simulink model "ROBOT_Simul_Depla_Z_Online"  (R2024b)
settings: Solver=ode15s  StartTime=0.0  StopTime=0.2  RelTol=1e-3  EnableMultiTasking=on
undefined symbols (not defined in the file): BATI1_Défaut_sldprt, BATI2_Défaut_sldprt, BATI3_Défaut_sldprt, BIELLE_Défaut_sldprt, BRAS_Défaut_sldprt, deg, Drive, EFFECTEUR_Défaut_sldprt, Fichiers, Fichiers_Matlab_sujetB, JOINT_Défaut_sldprt, kg, m, MANETTE_Défaut_sldprt, MATLAB, Matlab, mm, N, PIED_Défaut_sldprt, rad, s, STL, X, Y, Z
libraries: sm_lib x139, fl_lib x42, nesl_utility x19, slpidlib x3
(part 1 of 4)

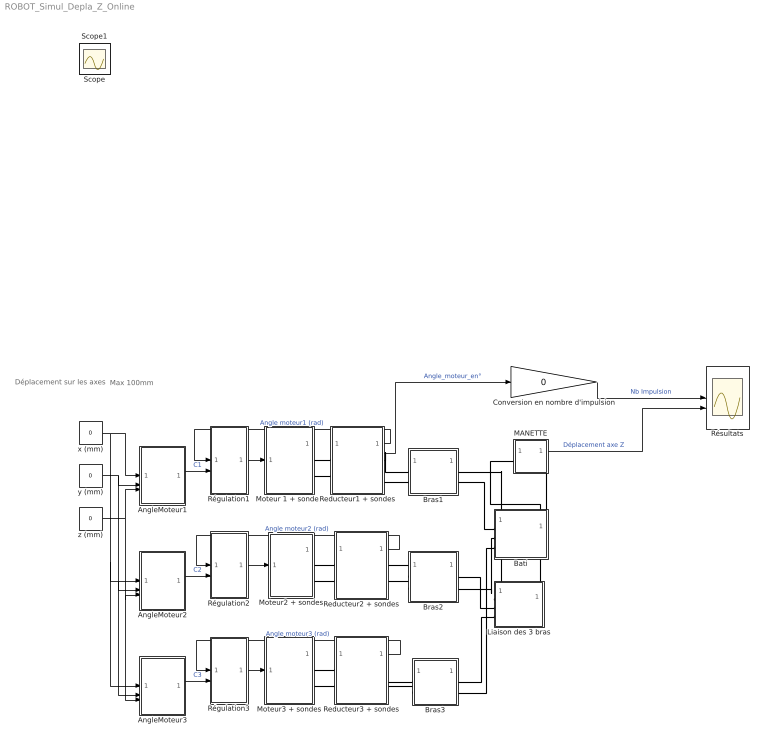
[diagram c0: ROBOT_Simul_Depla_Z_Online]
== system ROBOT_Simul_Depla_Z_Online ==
  note: Déplacement sur les axes
  note: Max 100mm
  AngleMoteur1 : MATLAB Function  TreatAsAtomicUnit=on
  AngleMoteur2 : MATLAB Function  TreatAsAtomicUnit=on
  AngleMoteur3 : MATLAB Function  TreatAsAtomicUnit=on
  Bati : Subsystem
  Bras1 : Subsystem
  Bras2 : Subsystem
  Bras3 : Subsystem
  Conversion en nombre d'impulsion : Gain  Gain=0
  Liaison des 3 bras : Subsystem
  MANETTE : Subsystem
  Moteur 1 + sondes : Subsystem
  Moteur2 + sondes : Subsystem
  Moteur3 + sondes : Subsystem
  Reducteur1 + sondes : Subsystem
  Reducteur2 + sondes : Subsystem
  Reducteur3 + sondes : Subsystem
  Régulation1 : Subsystem
  Régulation2 : Subsystem
  Régulation3 : Subsystem
  Résultats : Scope  NumInputPorts=2
  x (mm) : Constant  Value=0
  y (mm) : Constant  Value=0
  z (mm) : Constant  Value=0
  Scope : Scope
  Scope1 : Scope
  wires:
  Régulation3/1(Out1) -> Moteur3 + sondes/1(In1)
  Reducteur3 + sondes/1(Angle_mot3) -> Régulation3/1(In1)  "Angle moteur3 (rad)"
  Régulation1/1(Out1) -> Moteur 1 + sondes/1(In1)
  Reducteur1 + sondes/1(Angle_mot1) -> Régulation1/1(In1)  "Angle moteur1 (rad)"
  Régulation2/1(Out1) -> Moteur2 + sondes/1(In1)
  Reducteur2 + sondes/1(Angle_mot2) -> Régulation2/1(In1)  "Angle moteur2 (rad)"
  AngleMoteur3/1(anglmot3) -> Régulation3/2(In2)  "C3"
  x (mm)/1 -> AngleMoteur1/1(x), AngleMoteur2/1(x), AngleMoteur3/1(x)
  AngleMoteur1/1(anglmot1) -> Régulation1/2(In2)  "C1"
  AngleMoteur2/1(anglmot2) -> Régulation2/2(In2)  "C2"
  y (mm)/1 -> AngleMoteur1/2(y), AngleMoteur2/2(y), AngleMoteur3/2(y)
  z (mm)/1 -> AngleMoteur1/3(z), AngleMoteur2/3(z), AngleMoteur3/3(z)
  Reducteur1 + sondes/2(Angle_mot_°) -> Conversion en nombre d'impulsion/1  "Angle_moteur_en°"
  Conversion en nombre d'impulsion/1 -> Résultats/1  "Nb Impulsion"
  MANETTE/1(Out1) -> Résultats/2  "Déplacement axe Z"
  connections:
  Liaison des 3 bras/RConn1 -- MANETTE/LConn1
  Moteur3 + sondes/RConn1 -- Reducteur3 + sondes/LConn1
  Moteur 1 + sondes/RConn1 -- Reducteur1 + sondes/LConn1
  Moteur3 + sondes/RConn2 -- Reducteur3 + sondes/LConn2
  Reducteur1 + sondes/LConn2 -- Moteur 1 + sondes/RConn2
  Moteur2 + sondes/RConn2 -- Reducteur2 + sondes/LConn2
  Moteur2 + sondes/RConn1 -- Reducteur2 + sondes/LConn1
  Reducteur1 + sondes/RConn1 -- Bras1/LConn1
  Reducteur1 + sondes/RConn2 -- Bras1/LConn2
  Liaison des 3 bras/LConn1 -- Bras1/RConn1
  Liaison des 3 bras/LConn2 -- Bras2/RConn1
  Bras2/LConn1 -- Reducteur2 + sondes/RConn1
  Bras2/LConn2 -- Reducteur2 + sondes/RConn2
  Liaison des 3 bras/LConn3 -- Bras3/RConn1
  Reducteur3 + sondes/RConn1 -- Bras3/LConn1
  Bras3/LConn2 -- Reducteur3 + sondes/RConn2
  Bati/LConn1 -- Bras1/RConn2
  Bati/LConn2 -- Bras2/RConn2
  Bati/LConn3 -- Bras3/RConn2
  MANETTE/RConn1 -- Bati/RConn1

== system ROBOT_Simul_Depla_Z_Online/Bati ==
  BATI_1_RIGID : Subsystem
  MechanismConfiguration : sm_lib/Utilities/Mechanism Configuration  UniformGravity=Constant  GravityVector=[0 -9.81 0]  GravityVectorUnits=m/s^2  LinearizationDelta=0.001  JointModeTransitionNonlinearIterations=2
  Solver Configuration : nesl_utility/Solver Configuration  PhysicalDomain=network_engine_domain  SubClassName=solver  LeftPortType=input  RightPortType=generic  Tones=[]  Harmonics=[]  SimulateNoise=off  Profile=off  UseLocalSampling=off  EnableSwitchedLinearOptims=on  FrequencyDomain=off  UseCCode=off  RelTol=0.001  AbsTol=1e-06  MinStep=1e-09  ToWorkspace=off  RevertToSquareIcSolve=off  NumHomotopyIterations=100  PhasorMode=off  PhasorModeNumHarmonics=1  ConsistencySolver=NEWTON_FTOL  IndexReductionMethod=DerivativeReplacement  DoDC=off  ResidualTolerance=1e-09  ConsistencyTolSource=GLOBAL  ConsistencyAbsTol=0.001  ConsistencyRelTol=0.001  ConsistencyTolFactor=0.001  UseLocalSolver=off  LocalSolverChoice=NE_BACKWARD_EULER_ADVANCER  ResolveIndetEquations=on  FunctionEvalNumThread=1  LocalSolverSampleTime=0.001  DoFixedCost=off  MaxNonlinIter=3  MaxModeIter=2  ComputeImpulses=off  ImpulseIterations=2  LinearAlgebra=Sparse  LinearAlgebraNumThread=0  EquationFormulation=NE_TIME_EF  DelaysMemoryBudget=1024  AutomaticFiltering=on  FilteringTimeConstant=0.001  PartitionStorageMethod=AS_NEEDED  PartitionMemoryBudget=1024  PartitionMethod=FAST  MultibodyUseLocalSolver=off  MultibodyLocalSolverChoice=ODE1  MultibodyLocalSolverSampleTime=0.001
  Transform : sm_lib/Frames and Transforms/Rigid Transform  RotationMethod=ArbitraryAxis  FollAlignAxisA=+X  BaseAlignAxisA=+Y  FollAlignAxisB=+Y  BaseAlignAxisB=+Z  RotationStandardAxis=+Z  RotationAngle=1.8228218707828856  RotationAngleUnits=rad  RotationArbitraryAxis=[4.4011854841110467e-16 1.1162668393823967e-16 -1]  RotationSequenceAxes=FollowerAxes  RotationSequence=XYX  RotationSequenceAngles=[0 0 0]  RotationSequenceAnglesUnits=deg  RotationMatrix=[1 0 0; 0 1 0; 0 0 1]  Quaternion=[1 0 0 0]  TranslationMethod=Cartesian  TranslationCartesianOffset=[14.920329062241711 -30.551170260312524 -19.999999999988649]  TranslationCartesianOffsetUnits=mm  TranslationStandardAxis=+Z  TranslationStandardOffset=0  TranslationStandardOffsetUnits=mm  TranslationROffset=0  TranslationROffsetUnits=m  TranslationThetaOffset=0  TranslationThetaOffsetUnits=deg  TranslationZOffset=0  TranslationZOffsetUnits=m
  World : sm_lib/Frames and Transforms/World Frame
  E1 : PMIOPort  Side=Left
  E2 : PMIOPort  Port=2  Side=Left
  E3 : PMIOPort  Port=3  Side=Left
  Wrld : PMIOPort  Port=4  Side=Right
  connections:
  Transform/LConn1 -- MechanismConfiguration/RConn1 -- Wrld/RConn1 -- World/RConn1 -- Solver Configuration/RConn1
  BATI_1_RIGID/LConn1 -- Transform/RConn1
  BATI_1_RIGID/RConn3 -- E1/RConn1
  BATI_1_RIGID/RConn1 -- E3/RConn1
  BATI_1_RIGID/RConn2 -- E2/RConn1

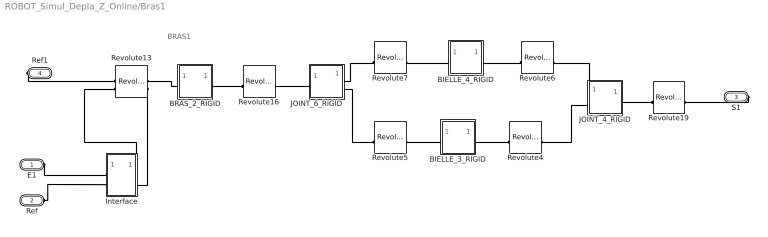
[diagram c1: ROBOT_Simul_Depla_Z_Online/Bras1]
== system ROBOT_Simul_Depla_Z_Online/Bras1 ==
  note: BRAS1
  BIELLE_3_RIGID : Subsystem
  BIELLE_4_RIGID : Subsystem
  BRAS_2_RIGID : Subsystem
  Interface : Subsystem
  JOINT_4_RIGID : Subsystem
  JOINT_6_RIGID : Subsystem
  Revolute13 : sm_lib/Joints/Revolute Joint  JointMode=Normal  CompositeWrenchDir=FollowerOnBase  CompositeWrenchFrame=BaseFrame  SenseConstraintForce=off  SenseConstraintTorque=off  SenseTotalForce=off  SenseTotalTorque=off  PositionTargetSpecify=on  PositionTargetPriority=Low  PositionTargetValue=11.887378711744704  PositionTargetValueUnits=deg  VelocityTargetSpecify=off  VelocityTargetPriority=High  VelocityTargetValue=0  VelocityTargetValueUnits=deg/s  EquilibriumPosition=0  EquilibriumPositionUnits=rad  SpringStiffness=0  SpringStiffnessUnits=m*N/rad  DampingCoefficient=0  DampingCoefficientUnits=m*s*N/rad  LowerLimitSpecify=off  LowerLimitBound=-90  LowerLimitBoundUnits=deg  LowerLimitStiffness=1e4  LowerLimitStiffnessUnits=N*m/deg  LowerLimitDamping=10  LowerLimitDampingUnits=N*m/(deg/s)  LowerLimitTransitionRegionWidth=0.1  LowerLimitTransitionRegionWidthUnits=deg  UpperLimitSpecify=off  UpperLimitBound=90  UpperLimitBoundUnits=deg  UpperLimitStiffness=1e4  UpperLimitStiffnessUnits=N*m/deg  UpperLimitDamping=10  UpperLimitDampingUnits=N*m/(deg/s)  UpperLimitTransitionRegionWidth=0.1  UpperLimitTransitionRegionWidthUnits=deg  TorqueActuationMode=InputTorque  MotionActuationMode=ComputedMotion  SensePosition=off  SenseVelocity=on  SenseAcceleration=off  SenseTorqueForce=off  SenseLowerLimitTorqueForce=off  SenseUpperLimitTorqueForce=off
  Revolute16 : sm_lib/Joints/Revolute Joint  JointMode=Normal  CompositeWrenchDir=FollowerOnBase  CompositeWrenchFrame=BaseFrame  SenseConstraintForce=off  SenseConstraintTorque=off  SenseTotalForce=off  SenseTotalTorque=off  PositionTargetSpecify=on  PositionTargetPriority=Low  PositionTargetValue=-127.14100786995047  PositionTargetValueUnits=deg  VelocityTargetSpecify=off  VelocityTargetPriority=High  VelocityTargetValue=0  VelocityTargetValueUnits=deg/s  EquilibriumPosition=0  EquilibriumPositionUnits=rad  SpringStiffness=0  SpringStiffnessUnits=m*N/rad  DampingCoefficient=0  DampingCoefficientUnits=m*s*N/rad  LowerLimitSpecify=off  LowerLimitBound=-90  LowerLimitBoundUnits=deg  LowerLimitStiffness=1e4  LowerLimitStiffnessUnits=N*m/deg  LowerLimitDamping=10  LowerLimitDampingUnits=N*m/(deg/s)  LowerLimitTransitionRegionWidth=0.1  LowerLimitTransitionRegionWidthUnits=deg  UpperLimitSpecify=off  UpperLimitBound=90  UpperLimitBoundUnits=deg  UpperLimitStiffness=1e4  UpperLimitStiffnessUnits=N*m/deg  UpperLimitDamping=10  UpperLimitDampingUnits=N*m/(deg/s)  UpperLimitTransitionRegionWidth=0.1  UpperLimitTransitionRegionWidthUnits=deg  TorqueActuationMode=NoTorque  MotionActuationMode=ComputedMotion  SensePosition=off  SenseVelocity=off  SenseAcceleration=off  SenseTorqueForce=off  SenseLowerLimitTorqueForce=off  SenseUpperLimitTorqueForce=off
  Revolute19 : sm_lib/Joints/Revolute Joint  JointMode=Normal  CompositeWrenchDir=FollowerOnBase  CompositeWrenchFrame=BaseFrame  SenseConstraintForce=off  SenseConstraintTorque=off  SenseTotalForce=off  SenseTotalTorque=off  PositionTargetSpecify=off  PositionTargetPriority=High  PositionTargetValue=0  PositionTargetValueUnits=deg  VelocityTargetSpecify=off  VelocityTargetPriority=High  VelocityTargetValue=0  VelocityTargetValueUnits=deg/s  EquilibriumPosition=0  EquilibriumPositionUnits=rad  SpringStiffness=0  SpringStiffnessUnits=m*N/rad  DampingCoefficient=0  DampingCoefficientUnits=m*s*N/rad  LowerLimitSpecify=off  LowerLimitBound=-90  LowerLimitBoundUnits=deg  LowerLimitStiffness=1e4  LowerLimitStiffnessUnits=N*m/deg  LowerLimitDamping=10  LowerLimitDampingUnits=N*m/(deg/s)  LowerLimitTransitionRegionWidth=0.1  LowerLimitTransitionRegionWidthUnits=deg  UpperLimitSpecify=off  UpperLimitBound=90  UpperLimitBoundUnits=deg  UpperLimitStiffness=1e4  UpperLimitStiffnessUnits=N*m/deg  UpperLimitDamping=10  UpperLimitDampingUnits=N*m/(deg/s)  UpperLimitTransitionRegionWidth=0.1  UpperLimitTransitionRegionWidthUnits=deg  TorqueActuationMode=NoTorque  MotionActuationMode=ComputedMotion  SensePosition=off  SenseVelocity=off  SenseAcceleration=off  SenseTorqueForce=off  SenseLowerLimitTorqueForce=off  SenseUpperLimitTorqueForce=off
  Revolute4 : sm_lib/Joints/Revolute Joint  JointMode=Normal  CompositeWrenchDir=FollowerOnBase  CompositeWrenchFrame=BaseFrame  SenseConstraintForce=off  SenseConstraintTorque=off  SenseTotalForce=off  SenseTotalTorque=off  PositionTargetSpecify=on  PositionTargetPriority=Low  PositionTargetValue=-91.30254308411611  PositionTargetValueUnits=deg  VelocityTargetSpecify=off  VelocityTargetPriority=High  VelocityTargetValue=0  VelocityTargetValueUnits=deg/s  EquilibriumPosition=0  EquilibriumPositionUnits=rad  SpringStiffness=0  SpringStiffnessUnits=m*N/rad  DampingCoefficient=0  DampingCoefficientUnits=m*s*N/rad  LowerLimitSpecify=off  LowerLimitBound=-90  LowerLimitBoundUnits=deg  LowerLimitStiffness=1e4  LowerLimitStiffnessUnits=N*m/deg  LowerLimitDamping=10  LowerLimitDampingUnits=N*m/(deg/s)  LowerLimitTransitionRegionWidth=0.1  LowerLimitTransitionRegionWidthUnits=deg  UpperLimitSpecify=off  UpperLimitBound=90  UpperLimitBoundUnits=deg  UpperLimitStiffness=1e4  UpperLimitStiffnessUnits=N*m/deg  UpperLimitDamping=10  UpperLimitDampingUnits=N*m/(deg/s)  UpperLimitTransitionRegionWidth=0.1  UpperLimitTransitionRegionWidthUnits=deg  TorqueActuationMode=NoTorque  MotionActuationMode=ComputedMotion  SensePosition=off  SenseVelocity=off  SenseAcceleration=off  SenseTorqueForce=off  SenseLowerLimitTorqueForce=off  SenseUpperLimitTorqueForce=off
  Revolute5 : sm_lib/Joints/Revolute Joint  JointMode=Normal  CompositeWrenchDir=FollowerOnBase  CompositeWrenchFrame=BaseFrame  SenseConstraintForce=off  SenseConstraintTorque=off  SenseTotalForce=off  SenseTotalTorque=off  PositionTargetSpecify=on  PositionTargetPriority=Low  PositionTargetValue=-91.302543084116394  PositionTargetValueUnits=deg  VelocityTargetSpecify=off  VelocityTargetPriority=High  VelocityTargetValue=0  VelocityTargetValueUnits=deg/s  EquilibriumPosition=0  EquilibriumPositionUnits=rad  SpringStiffness=0  SpringStiffnessUnits=m*N/rad  DampingCoefficient=0  DampingCoefficientUnits=m*s*N/rad  LowerLimitSpecify=off  LowerLimitBound=-90  LowerLimitBoundUnits=deg  LowerLimitStiffness=1e4  LowerLimitStiffnessUnits=N*m/deg  LowerLimitDamping=10  LowerLimitDampingUnits=N*m/(deg/s)  LowerLimitTransitionRegionWidth=0.1  LowerLimitTransitionRegionWidthUnits=deg  UpperLimitSpecify=off  UpperLimitBound=90  UpperLimitBoundUnits=deg  UpperLimitStiffness=1e4  UpperLimitStiffnessUnits=N*m/deg  UpperLimitDamping=10  UpperLimitDampingUnits=N*m/(deg/s)  UpperLimitTransitionRegionWidth=0.1  UpperLimitTransitionRegionWidthUnits=deg  TorqueActuationMode=NoTorque  MotionActuationMode=ComputedMotion  SensePosition=off  SenseVelocity=off  SenseAcceleration=off  SenseTorqueForce=off  SenseLowerLimitTorqueForce=off  SenseUpperLimitTorqueForce=off
  Revolute6 : sm_lib/Joints/Revolute Joint  JointMode=Normal  CompositeWrenchDir=FollowerOnBase  CompositeWrenchFrame=BaseFrame  SenseConstraintForce=off  SenseConstraintTorque=off  SenseTotalForce=off  SenseTotalTorque=off  PositionTargetSpecify=off  PositionTargetPriority=High  PositionTargetValue=0  PositionTargetValueUnits=deg  VelocityTargetSpecify=off  VelocityTargetPriority=High  VelocityTargetValue=0  VelocityTargetValueUnits=deg/s  EquilibriumPosition=0  EquilibriumPositionUnits=rad  SpringStiffness=0  SpringStiffnessUnits=m*N/rad  DampingCoefficient=0  DampingCoefficientUnits=m*s*N/rad  LowerLimitSpecify=off  LowerLimitBound=-90  LowerLimitBoundUnits=deg  LowerLimitStiffness=1e4  LowerLimitStiffnessUnits=N*m/deg  LowerLimitDamping=10  LowerLimitDampingUnits=N*m/(deg/s)  LowerLimitTransitionRegionWidth=0.1  LowerLimitTransitionRegionWidthUnits=deg  UpperLimitSpecify=off  UpperLimitBound=90  UpperLimitBoundUnits=deg  UpperLimitStiffness=1e4  UpperLimitStiffnessUnits=N*m/deg  UpperLimitDamping=10  UpperLimitDampingUnits=N*m/(deg/s)  UpperLimitTransitionRegionWidth=0.1  UpperLimitTransitionRegionWidthUnits=deg  TorqueActuationMode=NoTorque  MotionActuationMode=ComputedMotion  SensePosition=off  SenseVelocity=off  SenseAcceleration=off  SenseTorqueForce=off  SenseLowerLimitTorqueForce=off  SenseUpperLimitTorqueForce=off
  Revolute7 : sm_lib/Joints/Revolute Joint  JointMode=Normal  CompositeWrenchDir=FollowerOnBase  CompositeWrenchFrame=BaseFrame  SenseConstraintForce=off  SenseConstraintTorque=off  SenseTotalForce=off  SenseTotalTorque=off  PositionTargetSpecify=on  PositionTargetPriority=Low  PositionTargetValue=91.302543084116408  PositionTargetValueUnits=deg  VelocityTargetSpecify=off  VelocityTargetPriority=High  VelocityTargetValue=0  VelocityTargetValueUnits=deg/s  EquilibriumPosition=0  EquilibriumPositionUnits=rad  SpringStiffness=0  SpringStiffnessUnits=m*N/rad  DampingCoefficient=0  DampingCoefficientUnits=m*s*N/rad  LowerLimitSpecify=off  LowerLimitBound=-90  LowerLimitBoundUnits=deg  LowerLimitStiffness=1e4  LowerLimitStiffnessUnits=N*m/deg  LowerLimitDamping=10  LowerLimitDampingUnits=N*m/(deg/s)  LowerLimitTransitionRegionWidth=0.1  LowerLimitTransitionRegionWidthUnits=deg  UpperLimitSpecify=off  UpperLimitBound=90  UpperLimitBoundUnits=deg  UpperLimitStiffness=1e4  UpperLimitStiffnessUnits=N*m/deg  UpperLimitDamping=10  UpperLimitDampingUnits=N*m/(deg/s)  UpperLimitTransitionRegionWidth=0.1  UpperLimitTransitionRegionWidthUnits=deg  TorqueActuationMode=NoTorque  MotionActuationMode=ComputedMotion  SensePosition=off  SenseVelocity=off  SenseAcceleration=off  SenseTorqueForce=off  SenseLowerLimitTorqueForce=off  SenseUpperLimitTorqueForce=off
  E1 : PMIOPort  Side=Left
  Ref : PMIOPort  Port=2  Side=Left
  S1 : PMIOPort  Port=3  Side=Right
  Ref1 : PMIOPort  Port=4  Side=Right
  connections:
  JOINT_4_RIGID/LConn2 -- Revolute4/RConn1
  BIELLE_4_RIGID/LConn1 -- Revolute7/LConn1
  BIELLE_3_RIGID/LConn1 -- Revolute5/LConn1
  JOINT_6_RIGID/RConn2 -- Revolute5/RConn1
  BIELLE_4_RIGID/RConn1 -- Revolute6/LConn1
  JOINT_4_RIGID/LConn1 -- Revolute6/RConn1
  BRAS_2_RIGID/RConn1 -- Revolute16/LConn1
  S1/RConn1 -- Revolute19/LConn1
  BRAS_2_RIGID/LConn1 -- Revolute13/RConn1
  JOINT_4_RIGID/RConn1 -- Revolute19/RConn1
  JOINT_6_RIGID/LConn1 -- Revolute16/RConn1
  Ref1/RConn1 -- Revolute13/LConn1
  JOINT_6_RIGID/RConn1 -- Revolute7/RConn1
  BIELLE_3_RIGID/RConn1 -- Revolute4/LConn1
  Interface/RConn1 -- Revolute13/LConn2
  Interface/RConn2 -- Revolute13/RConn2
  E1/RConn1 -- Interface/LConn1
  Ref/RConn1 -- Interface/LConn2

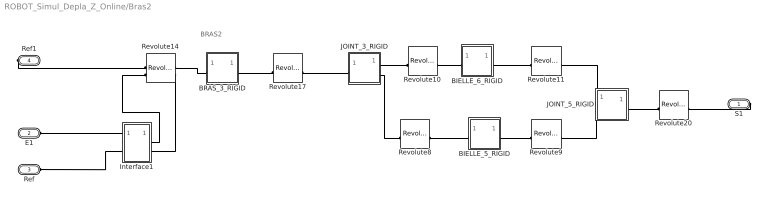
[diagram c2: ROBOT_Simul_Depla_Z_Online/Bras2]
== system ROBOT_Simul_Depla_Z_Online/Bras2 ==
  note: BRAS2
  BIELLE_5_RIGID : Subsystem
  BIELLE_6_RIGID : Subsystem
  BRAS_3_RIGID : Subsystem
  Interface1 : Subsystem
  JOINT_3_RIGID : Subsystem
  JOINT_5_RIGID : Subsystem
  Revolute10 : sm_lib/Joints/Revolute Joint  JointMode=Normal  CompositeWrenchDir=FollowerOnBase  CompositeWrenchFrame=BaseFrame  SenseConstraintForce=off  SenseConstraintTorque=off  SenseTotalForce=off  SenseTotalTorque=off  PositionTargetSpecify=on  PositionTargetPriority=Low  PositionTargetValue=-88.697456915883507  PositionTargetValueUnits=deg  VelocityTargetSpecify=off  VelocityTargetPriority=High  VelocityTargetValue=0  VelocityTargetValueUnits=deg/s  EquilibriumPosition=0  EquilibriumPositionUnits=rad  SpringStiffness=0  SpringStiffnessUnits=m*N/rad  DampingCoefficient=0  DampingCoefficientUnits=m*s*N/rad  LowerLimitSpecify=off  LowerLimitBound=-90  LowerLimitBoundUnits=deg  LowerLimitStiffness=1e4  LowerLimitStiffnessUnits=N*m/deg  LowerLimitDamping=10  LowerLimitDampingUnits=N*m/(deg/s)  LowerLimitTransitionRegionWidth=0.1  LowerLimitTransitionRegionWidthUnits=deg  UpperLimitSpecify=off  UpperLimitBound=90  UpperLimitBoundUnits=deg  UpperLimitStiffness=1e4  UpperLimitStiffnessUnits=N*m/deg  UpperLimitDamping=10  UpperLimitDampingUnits=N*m/(deg/s)  UpperLimitTransitionRegionWidth=0.1  UpperLimitTransitionRegionWidthUnits=deg  TorqueActuationMode=NoTorque  MotionActuationMode=ComputedMotion  SensePosition=off  SenseVelocity=off  SenseAcceleration=off  SenseTorqueForce=off  SenseLowerLimitTorqueForce=off  SenseUpperLimitTorqueForce=off
  Revolute11 : sm_lib/Joints/Revolute Joint  JointMode=Normal  CompositeWrenchDir=FollowerOnBase  CompositeWrenchFrame=BaseFrame  SenseConstraintForce=off  SenseConstraintTorque=off  SenseTotalForce=off  SenseTotalTorque=off  PositionTargetSpecify=off  PositionTargetPriority=High  PositionTargetValue=0  PositionTargetValueUnits=deg  VelocityTargetSpecify=off  VelocityTargetPriority=High  VelocityTargetValue=0  VelocityTargetValueUnits=deg/s  EquilibriumPosition=0  EquilibriumPositionUnits=rad  SpringStiffness=0  SpringStiffnessUnits=m*N/rad  DampingCoefficient=0  DampingCoefficientUnits=m*s*N/rad  LowerLimitSpecify=off  LowerLimitBound=-90  LowerLimitBoundUnits=deg  LowerLimitStiffness=1e4  LowerLimitStiffnessUnits=N*m/deg  LowerLimitDamping=10  LowerLimitDampingUnits=N*m/(deg/s)  LowerLimitTransitionRegionWidth=0.1  LowerLimitTransitionRegionWidthUnits=deg  UpperLimitSpecify=off  UpperLimitBound=90  UpperLimitBoundUnits=deg  UpperLimitStiffness=1e4  UpperLimitStiffnessUnits=N*m/deg  UpperLimitDamping=10  UpperLimitDampingUnits=N*m/(deg/s)  UpperLimitTransitionRegionWidth=0.1  UpperLimitTransitionRegionWidthUnits=deg  TorqueActuationMode=NoTorque  MotionActuationMode=ComputedMotion  SensePosition=off  SenseVelocity=off  SenseAcceleration=off  SenseTorqueForce=off  SenseLowerLimitTorqueForce=off  SenseUpperLimitTorqueForce=off
  Revolute14 : sm_lib/Joints/Revolute Joint  JointMode=Normal  CompositeWrenchDir=FollowerOnBase  CompositeWrenchFrame=BaseFrame  SenseConstraintForce=off  SenseConstraintTorque=off  SenseTotalForce=off  SenseTotalTorque=off  PositionTargetSpecify=on  PositionTargetPriority=Low  PositionTargetValue=-168.11262128825132  PositionTargetValueUnits=deg  VelocityTargetSpecify=off  VelocityTargetPriority=High  VelocityTargetValue=0  VelocityTargetValueUnits=deg/s  EquilibriumPosition=0  EquilibriumPositionUnits=rad  SpringStiffness=0  SpringStiffnessUnits=m*N/rad  DampingCoefficient=0  DampingCoefficientUnits=m*s*N/rad  LowerLimitSpecify=off  LowerLimitBound=-90  LowerLimitBoundUnits=deg  LowerLimitStiffness=1e4  LowerLimitStiffnessUnits=N*m/deg  LowerLimitDamping=10  LowerLimitDampingUnits=N*m/(deg/s)  LowerLimitTransitionRegionWidth=0.1  LowerLimitTransitionRegionWidthUnits=deg  UpperLimitSpecify=off  UpperLimitBound=90  UpperLimitBoundUnits=deg  UpperLimitStiffness=1e4  UpperLimitStiffnessUnits=N*m/deg  UpperLimitDamping=10  UpperLimitDampingUnits=N*m/(deg/s)  UpperLimitTransitionRegionWidth=0.1  UpperLimitTransitionRegionWidthUnits=deg  TorqueActuationMode=InputTorque  MotionActuationMode=ComputedMotion  SensePosition=off  SenseVelocity=on  SenseAcceleration=off  SenseTorqueForce=off  SenseLowerLimitTorqueForce=off  SenseUpperLimitTorqueForce=off
  Revolute17 : sm_lib/Joints/Revolute Joint  JointMode=Normal  CompositeWrenchDir=FollowerOnBase  CompositeWrenchFrame=BaseFrame  SenseConstraintForce=off  SenseConstraintTorque=off  SenseTotalForce=off  SenseTotalTorque=off  PositionTargetSpecify=on  PositionTargetPriority=Low  PositionTargetValue=-52.858992130053309  PositionTargetValueUnits=deg  VelocityTargetSpecify=off  VelocityTargetPriority=High  VelocityTargetValue=0  VelocityTargetValueUnits=deg/s  EquilibriumPosition=0  EquilibriumPositionUnits=rad  SpringStiffness=0  SpringStiffnessUnits=m*N/rad  DampingCoefficient=0  DampingCoefficientUnits=m*s*N/rad  LowerLimitSpecify=off  LowerLimitBound=-90  LowerLimitBoundUnits=deg  LowerLimitStiffness=1e4  LowerLimitStiffnessUnits=N*m/deg  LowerLimitDamping=10  LowerLimitDampingUnits=N*m/(deg/s)  LowerLimitTransitionRegionWidth=0.1  LowerLimitTransitionRegionWidthUnits=deg  UpperLimitSpecify=off  UpperLimitBound=90  UpperLimitBoundUnits=deg  UpperLimitStiffness=1e4  UpperLimitStiffnessUnits=N*m/deg  UpperLimitDamping=10  UpperLimitDampingUnits=N*m/(deg/s)  UpperLimitTransitionRegionWidth=0.1  UpperLimitTransitionRegionWidthUnits=deg  TorqueActuationMode=NoTorque  MotionActuationMode=ComputedMotion  SensePosition=off  SenseVelocity=off  SenseAcceleration=off  SenseTorqueForce=off  SenseLowerLimitTorqueForce=off  SenseUpperLimitTorqueForce=off
  Revolute20 : sm_lib/Joints/Revolute Joint  JointMode=Normal  CompositeWrenchDir=FollowerOnBase  CompositeWrenchFrame=BaseFrame  SenseConstraintForce=off  SenseConstraintTorque=off  SenseTotalForce=off  SenseTotalTorque=off  PositionTargetSpecify=off  PositionTargetPriority=High  PositionTargetValue=0  PositionTargetValueUnits=deg  VelocityTargetSpecify=off  VelocityTargetPriority=High  VelocityTargetValue=0  VelocityTargetValueUnits=deg/s  EquilibriumPosition=0  EquilibriumPositionUnits=rad  SpringStiffness=0  SpringStiffnessUnits=m*N/rad  DampingCoefficient=0  DampingCoefficientUnits=m*s*N/rad  LowerLimitSpecify=off  LowerLimitBound=-90  LowerLimitBoundUnits=deg  LowerLimitStiffness=1e4  LowerLimitStiffnessUnits=N*m/deg  LowerLimitDamping=10  LowerLimitDampingUnits=N*m/(deg/s)  LowerLimitTransitionRegionWidth=0.1  LowerLimitTransitionRegionWidthUnits=deg  UpperLimitSpecify=off  UpperLimitBound=90  UpperLimitBoundUnits=deg  UpperLimitStiffness=1e4  UpperLimitStiffnessUnits=N*m/deg  UpperLimitDamping=10  UpperLimitDampingUnits=N*m/(deg/s)  UpperLimitTransitionRegionWidth=0.1  UpperLimitTransitionRegionWidthUnits=deg  TorqueActuationMode=NoTorque  MotionActuationMode=ComputedMotion  SensePosition=off  SenseVelocity=off  SenseAcceleration=off  SenseTorqueForce=off  SenseLowerLimitTorqueForce=off  SenseUpperLimitTorqueForce=off
  Revolute8 : sm_lib/Joints/Revolute Joint  JointMode=Normal  CompositeWrenchDir=FollowerOnBase  CompositeWrenchFrame=BaseFrame  SenseConstraintForce=off  SenseConstraintTorque=off  SenseTotalForce=off  SenseTotalTorque=off  PositionTargetSpecify=on  PositionTargetPriority=Low  PositionTargetValue=-88.697456915883478  PositionTargetValueUnits=deg  VelocityTargetSpecify=off  VelocityTargetPriority=High  VelocityTargetValue=0  VelocityTargetValueUnits=deg/s  EquilibriumPosition=0  EquilibriumPositionUnits=rad  SpringStiffness=0  SpringStiffnessUnits=m*N/rad  DampingCoefficient=0  DampingCoefficientUnits=m*s*N/rad  LowerLimitSpecify=off  LowerLimitBound=-90  LowerLimitBoundUnits=deg  LowerLimitStiffness=1e4  LowerLimitStiffnessUnits=N*m/deg  LowerLimitDamping=10  LowerLimitDampingUnits=N*m/(deg/s)  LowerLimitTransitionRegionWidth=0.1  LowerLimitTransitionRegionWidthUnits=deg  UpperLimitSpecify=off  UpperLimitBound=90  UpperLimitBoundUnits=deg  UpperLimitStiffness=1e4  UpperLimitStiffnessUnits=N*m/deg  UpperLimitDamping=10  UpperLimitDampingUnits=N*m/(deg/s)  UpperLimitTransitionRegionWidth=0.1  UpperLimitTransitionRegionWidthUnits=deg  TorqueActuationMode=NoTorque  MotionActuationMode=ComputedMotion  SensePosition=off  SenseVelocity=off  SenseAcceleration=off  SenseTorqueForce=off  SenseLowerLimitTorqueForce=off  SenseUpperLimitTorqueForce=off
  Revolute9 : sm_lib/Joints/Revolute Joint  JointMode=Normal  CompositeWrenchDir=FollowerOnBase  CompositeWrenchFrame=BaseFrame  SenseConstraintForce=off  SenseConstraintTorque=off  SenseTotalForce=off  SenseTotalTorque=off  PositionTargetSpecify=on  PositionTargetPriority=Low  PositionTargetValue=91.30254308411601  PositionTargetValueUnits=deg  VelocityTargetSpecify=off  VelocityTargetPriority=High  VelocityTargetValue=0  VelocityTargetValueUnits=deg/s  EquilibriumPosition=0  EquilibriumPositionUnits=rad  SpringStiffness=0  SpringStiffnessUnits=m*N/rad  DampingCoefficient=0  DampingCoefficientUnits=m*s*N/rad  LowerLimitSpecify=off  LowerLimitBound=-90  LowerLimitBoundUnits=deg  LowerLimitStiffness=1e4  LowerLimitStiffnessUnits=N*m/deg  LowerLimitDamping=10  LowerLimitDampingUnits=N*m/(deg/s)  LowerLimitTransitionRegionWidth=0.1  LowerLimitTransitionRegionWidthUnits=deg  UpperLimitSpecify=off  UpperLimitBound=90  UpperLimitBoundUnits=deg  UpperLimitStiffness=1e4  UpperLimitStiffnessUnits=N*m/deg  UpperLimitDamping=10  UpperLimitDampingUnits=N*m/(deg/s)  UpperLimitTransitionRegionWidth=0.1  UpperLimitTransitionRegionWidthUnits=deg  TorqueActuationMode=NoTorque  MotionActuationMode=ComputedMotion  SensePosition=off  SenseVelocity=off  SenseAcceleration=off  SenseTorqueForce=off  SenseLowerLimitTorqueForce=off  SenseUpperLimitTorqueForce=off
  S1 : PMIOPort  Side=Right
  E1 : PMIOPort  Port=2  Side=Left
  Ref : PMIOPort  Port=3  Side=Left
  Ref1 : PMIOPort  Port=4  Side=Right
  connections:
  Interface1/RConn1 -- Revolute14/LConn2
  Interface1/LConn2 -- Ref/RConn1
  Interface1/RConn2 -- Revolute14/RConn2
  Interface1/LConn1 -- E1/RConn1
  BIELLE_5_RIGID/LConn1 -- Revolute8/LConn1
  BIELLE_6_RIGID/LConn1 -- Revolute10/LConn1
  JOINT_5_RIGID/LConn2 -- Revolute9/RConn1
  JOINT_3_RIGID/RConn1 -- Revolute10/RConn1
  JOINT_5_RIGID/LConn1 -- Revolute11/RConn1
  Ref1/RConn1 -- Revolute14/LConn1
  BRAS_3_RIGID/RConn1 -- Revolute17/LConn1
  BIELLE_5_RIGID/RConn1 -- Revolute9/LConn1
  JOINT_5_RIGID/RConn1 -- Revolute20/RConn1
  BIELLE_6_RIGID/RConn1 -- Revolute11/LConn1
  BRAS_3_RIGID/LConn1 -- Revolute14/RConn1
  S1/RConn1 -- Revolute20/LConn1
  JOINT_3_RIGID/RConn2 -- Revolute8/RConn1
  JOINT_3_RIGID/LConn1 -- Revolute17/RConn1

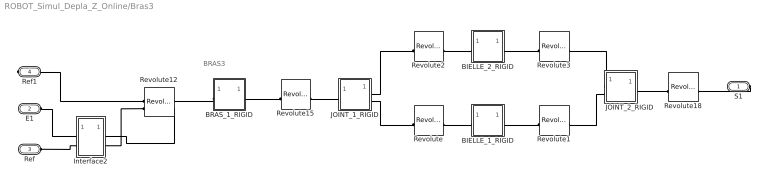
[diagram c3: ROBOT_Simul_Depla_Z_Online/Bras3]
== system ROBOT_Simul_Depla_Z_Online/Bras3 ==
  note: BRAS3
  BIELLE_1_RIGID : Subsystem
  BIELLE_2_RIGID : Subsystem
  BRAS_1_RIGID : Subsystem
  Interface2 : Subsystem
  JOINT_1_RIGID : Subsystem
  JOINT_2_RIGID : Subsystem
  Revolute : sm_lib/Joints/Revolute Joint  JointMode=Normal  CompositeWrenchDir=FollowerOnBase  CompositeWrenchFrame=BaseFrame  SenseConstraintForce=off  SenseConstraintTorque=off  SenseTotalForce=off  SenseTotalTorque=off  PositionTargetSpecify=on  PositionTargetPriority=Low  PositionTargetValue=91.302543084116763  PositionTargetValueUnits=deg  VelocityTargetSpecify=off  VelocityTargetPriority=High  VelocityTargetValue=0  VelocityTargetValueUnits=deg/s  EquilibriumPosition=0  EquilibriumPositionUnits=rad  SpringStiffness=0  SpringStiffnessUnits=m*N/rad  DampingCoefficient=0  DampingCoefficientUnits=m*s*N/rad  LowerLimitSpecify=off  LowerLimitBound=-90  LowerLimitBoundUnits=deg  LowerLimitStiffness=1e4  LowerLimitStiffnessUnits=N*m/deg  LowerLimitDamping=10  LowerLimitDampingUnits=N*m/(deg/s)  LowerLimitTransitionRegionWidth=0.1  LowerLimitTransitionRegionWidthUnits=deg  UpperLimitSpecify=off  UpperLimitBound=90  UpperLimitBoundUnits=deg  UpperLimitStiffness=1e4  UpperLimitStiffnessUnits=N*m/deg  UpperLimitDamping=10  UpperLimitDampingUnits=N*m/(deg/s)  UpperLimitTransitionRegionWidth=0.1  UpperLimitTransitionRegionWidthUnits=deg  TorqueActuationMode=NoTorque  MotionActuationMode=ComputedMotion  SensePosition=off  SenseVelocity=off  SenseAcceleration=off  SenseTorqueForce=off  SenseLowerLimitTorqueForce=off  SenseUpperLimitTorqueForce=off
  Revolute1 : sm_lib/Joints/Revolute Joint  JointMode=Normal  CompositeWrenchDir=FollowerOnBase  CompositeWrenchFrame=BaseFrame  SenseConstraintForce=off  SenseConstraintTorque=off  SenseTotalForce=off  SenseTotalTorque=off  PositionTargetSpecify=on  PositionTargetPriority=Low  PositionTargetValue=91.302543084117588  PositionTargetValueUnits=deg  VelocityTargetSpecify=off  VelocityTargetPriority=High  VelocityTargetValue=0  VelocityTargetValueUnits=deg/s  EquilibriumPosition=0  EquilibriumPositionUnits=rad  SpringStiffness=0  SpringStiffnessUnits=m*N/rad  DampingCoefficient=0  DampingCoefficientUnits=m*s*N/rad  LowerLimitSpecify=off  LowerLimitBound=-90  LowerLimitBoundUnits=deg  LowerLimitStiffness=1e4  LowerLimitStiffnessUnits=N*m/deg  LowerLimitDamping=10  LowerLimitDampingUnits=N*m/(deg/s)  LowerLimitTransitionRegionWidth=0.1  LowerLimitTransitionRegionWidthUnits=deg  UpperLimitSpecify=off  UpperLimitBound=90  UpperLimitBoundUnits=deg  UpperLimitStiffness=1e4  UpperLimitStiffnessUnits=N*m/deg  UpperLimitDamping=10  UpperLimitDampingUnits=N*m/(deg/s)  UpperLimitTransitionRegionWidth=0.1  UpperLimitTransitionRegionWidthUnits=deg  TorqueActuationMode=NoTorque  MotionActuationMode=ComputedMotion  SensePosition=off  SenseVelocity=off  SenseAcceleration=off  SenseTorqueForce=off  SenseLowerLimitTorqueForce=off  SenseUpperLimitTorqueForce=off
  Revolute12 : sm_lib/Joints/Revolute Joint  JointMode=Normal  CompositeWrenchDir=FollowerOnBase  CompositeWrenchFrame=BaseFrame  SenseConstraintForce=off  SenseConstraintTorque=off  SenseTotalForce=off  SenseTotalTorque=off  PositionTargetSpecify=on  PositionTargetPriority=Low  PositionTargetValue=-101.88737871174806  PositionTargetValueUnits=deg  VelocityTargetSpecify=off  VelocityTargetPriority=High  VelocityTargetValue=0  VelocityTargetValueUnits=deg/s  EquilibriumPosition=0  EquilibriumPositionUnits=rad  SpringStiffness=0  SpringStiffnessUnits=m*N/rad  DampingCoefficient=0  DampingCoefficientUnits=m*s*N/rad  LowerLimitSpecify=off  LowerLimitBound=-90  LowerLimitBoundUnits=deg  LowerLimitStiffness=1e4  LowerLimitStiffnessUnits=N*m/deg  LowerLimitDamping=10  LowerLimitDampingUnits=N*m/(deg/s)  LowerLimitTransitionRegionWidth=0.1  LowerLimitTransitionRegionWidthUnits=deg  UpperLimitSpecify=off  UpperLimitBound=90  UpperLimitBoundUnits=deg  UpperLimitStiffness=1e4  UpperLimitStiffnessUnits=N*m/deg  UpperLimitDamping=10  UpperLimitDampingUnits=N*m/(deg/s)  UpperLimitTransitionRegionWidth=0.1  UpperLimitTransitionRegionWidthUnits=deg  TorqueActuationMode=InputTorque  MotionActuationMode=ComputedMotion  SensePosition=off  SenseVelocity=on  SenseAcceleration=off  SenseTorqueForce=off  SenseLowerLimitTorqueForce=off  SenseUpperLimitTorqueForce=off
  Revolute15 : sm_lib/Joints/Revolute Joint  JointMode=Normal  CompositeWrenchDir=FollowerOnBase  CompositeWrenchFrame=BaseFrame  SenseConstraintForce=off  SenseConstraintTorque=off  SenseTotalForce=off  SenseTotalTorque=off  PositionTargetSpecify=on  PositionTargetPriority=Low  PositionTargetValue=-52.858992130052194  PositionTargetValueUnits=deg  VelocityTargetSpecify=off  VelocityTargetPriority=High  VelocityTargetValue=0  VelocityTargetValueUnits=deg/s  EquilibriumPosition=0  EquilibriumPositionUnits=rad  SpringStiffness=0  SpringStiffnessUnits=m*N/rad  DampingCoefficient=0  DampingCoefficientUnits=m*s*N/rad  LowerLimitSpecify=off  LowerLimitBound=-90  LowerLimitBoundUnits=deg  LowerLimitStiffness=1e4  LowerLimitStiffnessUnits=N*m/deg  LowerLimitDamping=10  LowerLimitDampingUnits=N*m/(deg/s)  LowerLimitTransitionRegionWidth=0.1  LowerLimitTransitionRegionWidthUnits=deg  UpperLimitSpecify=off  UpperLimitBound=90  UpperLimitBoundUnits=deg  UpperLimitStiffness=1e4  UpperLimitStiffnessUnits=N*m/deg  UpperLimitDamping=10  UpperLimitDampingUnits=N*m/(deg/s)  UpperLimitTransitionRegionWidth=0.1  UpperLimitTransitionRegionWidthUnits=deg  TorqueActuationMode=NoTorque  MotionActuationMode=ComputedMotion  SensePosition=off  SenseVelocity=off  SenseAcceleration=off  SenseTorqueForce=off  SenseLowerLimitTorqueForce=off  SenseUpperLimitTorqueForce=off
  Revolute18 : sm_lib/Joints/Revolute Joint  JointMode=Normal  CompositeWrenchDir=FollowerOnBase  CompositeWrenchFrame=BaseFrame  SenseConstraintForce=off  SenseConstraintTorque=off  SenseTotalForce=off  SenseTotalTorque=off  PositionTargetSpecify=on  PositionTargetPriority=Low  PositionTargetValue=-139.02838658169591  PositionTargetValueUnits=deg  VelocityTargetSpecify=off  VelocityTargetPriority=High  VelocityTargetValue=0  VelocityTargetValueUnits=deg/s  EquilibriumPosition=0  EquilibriumPositionUnits=rad  SpringStiffness=0  SpringStiffnessUnits=m*N/rad  DampingCoefficient=0  DampingCoefficientUnits=m*s*N/rad  LowerLimitSpecify=off  LowerLimitBound=-90  LowerLimitBoundUnits=deg  LowerLimitStiffness=1e4  LowerLimitStiffnessUnits=N*m/deg  LowerLimitDamping=10  LowerLimitDampingUnits=N*m/(deg/s)  LowerLimitTransitionRegionWidth=0.1  LowerLimitTransitionRegionWidthUnits=deg  UpperLimitSpecify=off  UpperLimitBound=90  UpperLimitBoundUnits=deg  UpperLimitStiffness=1e4  UpperLimitStiffnessUnits=N*m/deg  UpperLimitDamping=10  UpperLimitDampingUnits=N*m/(deg/s)  UpperLimitTransitionRegionWidth=0.1  UpperLimitTransitionRegionWidthUnits=deg  TorqueActuationMode=NoTorque  MotionActuationMode=ComputedMotion  SensePosition=off  SenseVelocity=off  SenseAcceleration=off  SenseTorqueForce=off  SenseLowerLimitTorqueForce=off  SenseUpperLimitTorqueForce=off
  Revolute2 : sm_lib/Joints/Revolute Joint  JointMode=Normal  CompositeWrenchDir=FollowerOnBase  CompositeWrenchFrame=BaseFrame  SenseConstraintForce=off  SenseConstraintTorque=off  SenseTotalForce=off  SenseTotalTorque=off  PositionTargetSpecify=on  PositionTargetPriority=Low  PositionTargetValue=-88.697456915883265  PositionTargetValueUnits=deg  VelocityTargetSpecify=off  VelocityTargetPriority=High  VelocityTargetValue=0  VelocityTargetValueUnits=deg/s  EquilibriumPosition=0  EquilibriumPositionUnits=rad  SpringStiffness=0  SpringStiffnessUnits=m*N/rad  DampingCoefficient=0  DampingCoefficientUnits=m*s*N/rad  LowerLimitSpecify=off  LowerLimitBound=-90  LowerLimitBoundUnits=deg  LowerLimitStiffness=1e4  LowerLimitStiffnessUnits=N*m/deg  LowerLimitDamping=10  LowerLimitDampingUnits=N*m/(deg/s)  LowerLimitTransitionRegionWidth=0.1  LowerLimitTransitionRegionWidthUnits=deg  UpperLimitSpecify=off  UpperLimitBound=90  UpperLimitBoundUnits=deg  UpperLimitStiffness=1e4  UpperLimitStiffnessUnits=N*m/deg  UpperLimitDamping=10  UpperLimitDampingUnits=N*m/(deg/s)  UpperLimitTransitionRegionWidth=0.1  UpperLimitTransitionRegionWidthUnits=deg  TorqueActuationMode=NoTorque  MotionActuationMode=ComputedMotion  SensePosition=off  SenseVelocity=off  SenseAcceleration=off  SenseTorqueForce=off  SenseLowerLimitTorqueForce=off  SenseUpperLimitTorqueForce=off
  Revolute3 : sm_lib/Joints/Revolute Joint  JointMode=Normal  CompositeWrenchDir=FollowerOnBase  CompositeWrenchFrame=BaseFrame  SenseConstraintForce=off  SenseConstraintTorque=off  SenseTotalForce=off  SenseTotalTorque=off  PositionTargetSpecify=off  PositionTargetPriority=High  PositionTargetValue=0  PositionTargetValueUnits=deg  VelocityTargetSpecify=off  VelocityTargetPriority=High  VelocityTargetValue=0  VelocityTargetValueUnits=deg/s  EquilibriumPosition=0  EquilibriumPositionUnits=rad  SpringStiffness=0  SpringStiffnessUnits=m*N/rad  DampingCoefficient=0  DampingCoefficientUnits=m*s*N/rad  LowerLimitSpecify=off  LowerLimitBound=-90  LowerLimitBoundUnits=deg  LowerLimitStiffness=1e4  LowerLimitStiffnessUnits=N*m/deg  LowerLimitDamping=10  LowerLimitDampingUnits=N*m/(deg/s)  LowerLimitTransitionRegionWidth=0.1  LowerLimitTransitionRegionWidthUnits=deg  UpperLimitSpecify=off  UpperLimitBound=90  UpperLimitBoundUnits=deg  UpperLimitStiffness=1e4  UpperLimitStiffnessUnits=N*m/deg  UpperLimitDamping=10  UpperLimitDampingUnits=N*m/(deg/s)  UpperLimitTransitionRegionWidth=0.1  UpperLimitTransitionRegionWidthUnits=deg  TorqueActuationMode=NoTorque  MotionActuationMode=ComputedMotion  SensePosition=off  SenseVelocity=off  SenseAcceleration=off  SenseTorqueForce=off  SenseLowerLimitTorqueForce=off  SenseUpperLimitTorqueForce=off
  S1 : PMIOPort  Side=Right
  E1 : PMIOPort  Port=2  Side=Left
  Ref : PMIOPort  Port=3  Side=Left
  Ref1 : PMIOPort  Port=4  Side=Right
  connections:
  JOINT_1_RIGID/RConn2 -- Revolute/LConn1
  BRAS_1_RIGID/RConn1 -- Revolute15/LConn1
  Ref1/RConn1 -- Revolute12/RConn1
  S1/RConn1 -- Revolute18/RConn1
  JOINT_1_RIGID/LConn1 -- Revolute15/RConn1
  BIELLE_1_RIGID/LConn1 -- Revolute/RConn1
  BIELLE_1_RIGID/RConn1 -- Revolute1/LConn1
  BRAS_1_RIGID/LConn1 -- Revolute12/LConn1
  JOINT_2_RIGID/RConn1 -- Revolute18/LConn1
  JOINT_2_RIGID/LConn2 -- Revolute1/RConn1
  BIELLE_2_RIGID/LConn1 -- Revolute2/RConn1
  JOINT_1_RIGID/RConn1 -- Revolute2/LConn1
  JOINT_2_RIGID/LConn1 -- Revolute3/RConn1
  BIELLE_2_RIGID/RConn1 -- Revolute3/LConn1
  Interface2/LConn2 -- Ref/RConn1
  Interface2/RConn2 -- Revolute12/RConn2
  Interface2/RConn1 -- Revolute12/LConn2
  E1/RConn1 -- Interface2/LConn1

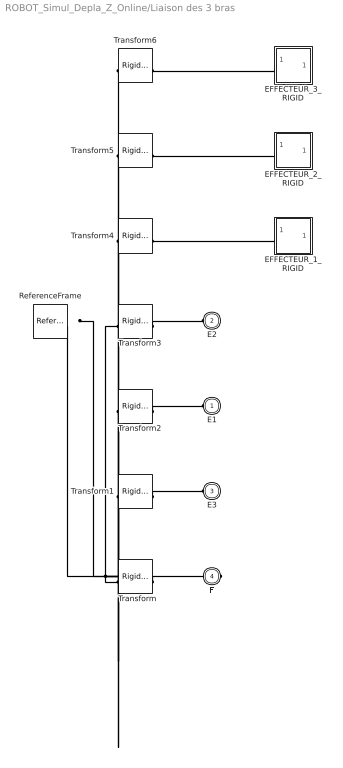
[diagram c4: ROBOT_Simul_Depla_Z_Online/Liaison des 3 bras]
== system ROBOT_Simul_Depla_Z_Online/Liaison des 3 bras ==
  EFFECTEUR_1_RIGID : Subsystem
  EFFECTEUR_2_RIGID : Subsystem
  EFFECTEUR_3_RIGID : Subsystem
  ReferenceFrame : sm_lib/Frames and Transforms/Reference Frame
  Transform : sm_lib/Frames and Transforms/Rigid Transform  RotationMethod=ArbitraryAxis  FollAlignAxisA=+X  BaseAlignAxisA=+Y  FollAlignAxisB=+Y  BaseAlignAxisB=+Z  RotationStandardAxis=+Z  RotationAngle=3.1415926535897931  RotationAngleUnits=rad  RotationArbitraryAxis=[1 0 0]  RotationSequenceAxes=FollowerAxes  RotationSequence=XYX  RotationSequenceAngles=[0 0 0]  RotationSequenceAnglesUnits=deg  RotationMatrix=[1 0 0; 0 1 0; 0 0 1]  Quaternion=[1 0 0 0]  TranslationMethod=Cartesian  TranslationCartesianOffset=[0 0 -32.350000000009082]  TranslationCartesianOffsetUnits=mm  TranslationStandardAxis=+Z  TranslationStandardOffset=0  TranslationStandardOffsetUnits=mm  TranslationROffset=0  TranslationROffsetUnits=m  TranslationThetaOffset=0  TranslationThetaOffsetUnits=deg  TranslationZOffset=0  TranslationZOffsetUnits=m
  Transform1 : sm_lib/Frames and Transforms/Rigid Transform  RotationMethod=ArbitraryAxis  FollAlignAxisA=+X  BaseAlignAxisA=+Y  FollAlignAxisB=+Y  BaseAlignAxisB=+Z  RotationStandardAxis=+Z  RotationAngle=2.4188584057763762  RotationAngleUnits=rad  RotationArbitraryAxis=[-0.65465367070797653 -0.37796447300922748 -0.65465367070797764]  RotationSequenceAxes=FollowerAxes  RotationSequence=XYX  RotationSequenceAngles=[0 0 0]  RotationSequenceAnglesUnits=deg  RotationMatrix=[1 0 0; 0 1 0; 0 0 1]  Quaternion=[1 0 0 0]  TranslationMethod=Cartesian  TranslationCartesianOffset=[-19.120111238677367 -12.995546039657871 14.999999999991132]  TranslationCartesianOffsetUnits=mm  TranslationStandardAxis=+Z  TranslationStandardOffset=0  TranslationStandardOffsetUnits=mm  TranslationROffset=0  TranslationROffsetUnits=m  TranslationThetaOffset=0  TranslationThetaOffsetUnits=deg  TranslationZOffset=0  TranslationZOffsetUnits=m
  Transform2 : sm_lib/Frames and Transforms/Rigid Transform  RotationMethod=ArbitraryAxis  FollAlignAxisA=+X  BaseAlignAxisA=+Y  FollAlignAxisB=+Y  BaseAlignAxisB=+Z  RotationStandardAxis=+Z  RotationAngle=2.4188584057763851  RotationAngleUnits=rad  RotationArbitraryAxis=[0.65465367070797842 -0.37796447300922287 0.65465367070797842]  RotationSequenceAxes=FollowerAxes  RotationSequence=XYX  RotationSequenceAngles=[0 0 0]  RotationSequenceAnglesUnits=deg  RotationMatrix=[1 0 0; 0 1 0; 0 0 1]  Quaternion=[1 0 0 0]  TranslationMethod=Cartesian  TranslationCartesianOffset=[2.6286000672859817 43.296105206329507 14.999999999990896]  TranslationCartesianOffsetUnits=mm  TranslationStandardAxis=+Z  TranslationStandardOffset=0  TranslationStandardOffsetUnits=mm  TranslationROffset=0  TranslationROffsetUnits=m  TranslationThetaOffset=0  TranslationThetaOffsetUnits=deg  TranslationZOffset=0  TranslationZOffsetUnits=m
  Transform3 : sm_lib/Frames and Transforms/Rigid Transform  RotationMethod=ArbitraryAxis  FollAlignAxisA=+X  BaseAlignAxisA=+Y  FollAlignAxisB=+Y  BaseAlignAxisB=+Z  RotationStandardAxis=+Z  RotationAngle=2.0943951023931993  RotationAngleUnits=rad  RotationArbitraryAxis=[-0.57735026918962318 -0.57735026918962706 0.57735026918962695]  RotationSequenceAxes=FollowerAxes  RotationSequence=XYX  RotationSequenceAngles=[0 0 0]  RotationSequenceAnglesUnits=deg  RotationMatrix=[1 0 0; 0 1 0; 0 0 1]  Quaternion=[1 0 0 0]  TranslationMethod=Cartesian  TranslationCartesianOffset=[43.004244414304381 -8.0147839261255491 14.99999999999091]  TranslationCartesianOffsetUnits=mm  TranslationStandardAxis=+Z  TranslationStandardOffset=0  TranslationStandardOffsetUnits=mm  TranslationROffset=0  TranslationROffsetUnits=m  TranslationThetaOffset=0  TranslationThetaOffsetUnits=deg  TranslationZOffset=0  TranslationZOffsetUnits=m
  Transform4 : sm_lib/Frames and Transforms/Rigid Transform  RotationMethod=None  FollAlignAxisA=+X  BaseAlignAxisA=+Y  FollAlignAxisB=+Y  BaseAlignAxisB=+Z  RotationStandardAxis=+Z  RotationAngle=0  RotationAngleUnits=deg  RotationArbitraryAxis=[0 0 1]  RotationSequenceAxes=FollowerAxes  RotationSequence=XYX  RotationSequenceAngles=[0 0 0]  RotationSequenceAnglesUnits=deg  RotationMatrix=[1 0 0; 0 1 0; 0 0 1]  Quaternion=[1 0 0 0]  TranslationMethod=Cartesian  TranslationCartesianOffset=[8.0042444143042797 5.9852160738742057 -9.0899510141184692e-12]  TranslationCartesianOffsetUnits=mm  TranslationStandardAxis=+Z  TranslationStandardOffset=0  TranslationStandardOffsetUnits=mm  TranslationROffset=0  TranslationROffsetUnits=m  TranslationThetaOffset=0  TranslationThetaOffsetUnits=deg  TranslationZOffset=0  TranslationZOffsetUnits=m
  Transform5 : sm_lib/Frames and Transforms/Rigid Transform  RotationMethod=ArbitraryAxis  FollAlignAxisA=+X  BaseAlignAxisA=+Y  FollAlignAxisB=+Y  BaseAlignAxisB=+Z  RotationStandardAxis=+Z  RotationAngle=2.0943951023932001  RotationAngleUnits=rad  RotationArbitraryAxis=[0 0 1]  RotationSequenceAxes=FollowerAxes  RotationSequence=XYX  RotationSequenceAngles=[0 0 0]  RotationSequenceAnglesUnits=deg  RotationMatrix=[1 0 0; 0 1 0; 0 0 1]  Quaternion=[1 0 0 0]  TranslationMethod=Cartesian  TranslationCartesianOffset=[8.0042444143042797 5.9852160738742057 -9.0899510141184692e-12]  TranslationCartesianOffsetUnits=mm  TranslationStandardAxis=+Z  TranslationStandardOffset=0  TranslationStandardOffsetUnits=mm  TranslationROffset=0  TranslationROffsetUnits=m  TranslationThetaOffset=0  TranslationThetaOffsetUnits=deg  TranslationZOffset=0  TranslationZOffsetUnits=m
  Transform6 : sm_lib/Frames and Transforms/Rigid Transform  RotationMethod=ArbitraryAxis  FollAlignAxisA=+X  BaseAlignAxisA=+Y  FollAlignAxisB=+Y  BaseAlignAxisB=+Z  RotationStandardAxis=+Z  RotationAngle=2.0943951023931859  RotationAngleUnits=rad  RotationArbitraryAxis=[-0 -0 -1]  RotationSequenceAxes=FollowerAxes  RotationSequence=XYX  RotationSequenceAngles=[0 0 0]  RotationSequenceAnglesUnits=deg  RotationMatrix=[1 0 0; 0 1 0; 0 0 1]  Quaternion=[1 0 0 0]  TranslationMethod=Cartesian  TranslationCartesianOffset=[8.0042444143042797 5.9852160738742057 -9.0899510141184692e-12]  TranslationCartesianOffsetUnits=mm  TranslationStandardAxis=+Z  TranslationStandardOffset=0  TranslationStandardOffsetUnits=mm  TranslationROffset=0  TranslationROffsetUnits=m  TranslationThetaOffset=0  TranslationThetaOffsetUnits=deg  TranslationZOffset=0  TranslationZOffsetUnits=m
  E1 : PMIOPort  Side=Left
  E2 : PMIOPort  Port=2  Side=Left
  E3 : PMIOPort  Port=3  Side=Left
  F : PMIOPort  Port=4  Side=Right
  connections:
  Transform/LConn1 -- ReferenceFrame/RConn1 -- Transform1/LConn1 -- Transform2/LConn1 -- Transform3/LConn1 -- Transform4/LConn1 -- Transform5/LConn1 -- Transform6/LConn1
  Transform/RConn1 -- F/RConn1
  Transform1/RConn1 -- E3/RConn1
  Transform2/RConn1 -- E1/RConn1
  Transform3/RConn1 -- E2/RConn1
  EFFECTEUR_1_RIGID/LConn1 -- Transform4/RConn1
  EFFECTEUR_2_RIGID/LConn1 -- Transform5/RConn1
  EFFECTEUR_3_RIGID/LConn1 -- Transform6/RConn1

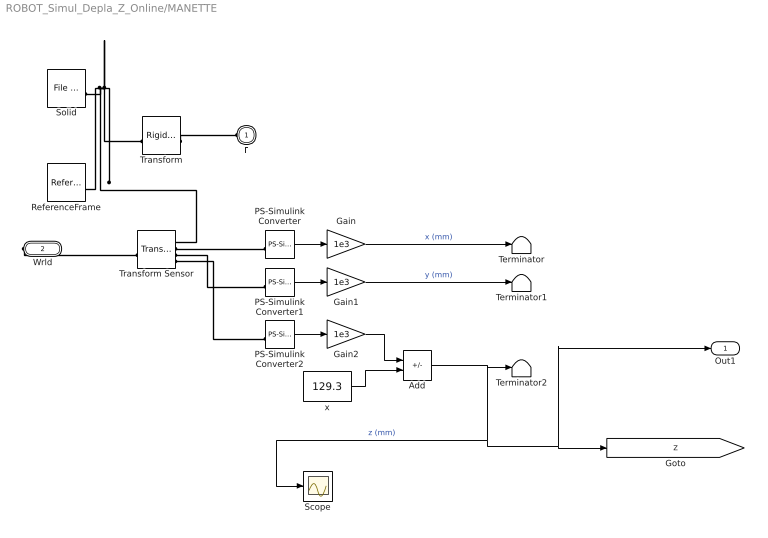
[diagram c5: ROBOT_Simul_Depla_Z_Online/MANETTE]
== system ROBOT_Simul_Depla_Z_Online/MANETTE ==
  Add : Sum  Inputs=+-
  Gain : Gain  Gain=1e3
  Gain1 : Gain  Gain=1e3
  Gain2 : Gain  Gain=1e3
  PS-Simulink Converter : nesl_utility/PS-Simulink Converter  PhysicalDomain=network_engine_domain  SubClassName=ps_output  LeftPortType=input  RightPortType=output  PseudoPeriodic=off  Frequencies=[]  VectorFormat=1-D array  Unit=1  AffineConversion=off
  PS-Simulink Converter1 : nesl_utility/PS-Simulink Converter  PhysicalDomain=network_engine_domain  SubClassName=ps_output  LeftPortType=input  RightPortType=output  PseudoPeriodic=off  Frequencies=[]  VectorFormat=1-D array  Unit=1  AffineConversion=off
  PS-Simulink Converter2 : nesl_utility/PS-Simulink Converter  PhysicalDomain=network_engine_domain  SubClassName=ps_output  LeftPortType=input  RightPortType=output  PseudoPeriodic=off  Frequencies=[]  VectorFormat=1-D array  Unit=1  AffineConversion=off
  ReferenceFrame : sm_lib/Frames and Transforms/Reference Frame
  Scope : Scope
  Solid : sm_lib/Body Elements/File Solid  ExtGeomFileName=/MATLAB Drive/Fichiers_Matlab_sujetB/Fichiers Matlab/STL/MANETTE_Défaut_sldprt.STL  UnitType=Custom  ExtGeomFileUnits=mm  StepReaderType=HEX  ExportConvexHullGeometry=off  InertiaType=Custom  BasedOnType=Density  Density=1000  DensityUnits=kg/(m^3)  Mass=0.040615337241087436  MassUnits=kg  CenterOfMass=[0 0.040047984959972249 0]  CenterOfMassUnits=mm  MomentsOfInertia=[8.2576276174464649 8.2126567442848692 8.2576263457676724]  MomentsOfInertiaUnits=kg*mm^2  ProductsOfInertia=[0 0 0]  ProductsOfInertiaUnits=kg*mm^2  GraphicType=FromGeometry  MarkerShape=Sphere  MarkerSize=10  GraphicVisPropType=SimpleVisualProperties  GraphicDiffuseColor=[0.69803921568627447 0.69803921568627447 0.69803921568627447]  GraphicOpacity=1  GraphicSpecularColor=[0.5 0.5 0.5 1.0]  GraphicAmbientColor=[0.15 0.15 0.15 1.0]  GraphicEmissiveColor=[0.0 0.0 0.0 1.0]  GraphicShininess=75  DoExposeReferenceFrame=on  SerializedFrames=<Frames/>
  Terminator : Terminator
  Terminator1 : Terminator
  Terminator2 : Terminator
  Transform : sm_lib/Frames and Transforms/Rigid Transform  RotationMethod=ArbitraryAxis  FollAlignAxisA=+X  BaseAlignAxisA=+Y  FollAlignAxisB=+Y  BaseAlignAxisB=+Z  RotationStandardAxis=+Z  RotationAngle=1.570796326794897  RotationAngleUnits=rad  RotationArbitraryAxis=[1 -1.5700924586837747e-16 -7.5435830438090697e-17]  RotationSequenceAxes=FollowerAxes  RotationSequence=XYX  RotationSequenceAngles=[0 0 0]  RotationSequenceAnglesUnits=deg  RotationMatrix=[1 0 0; 0 1 0; 0 0 1]  Quaternion=[1 0 0 0]  TranslationMethod=Cartesian  TranslationCartesianOffset=[-8.0042444143042815 2.4868995751603507e-14 5.9852160738742031]  TranslationCartesianOffsetUnits=mm  TranslationStandardAxis=+Z  TranslationStandardOffset=0  TranslationStandardOffsetUnits=mm  TranslationROffset=0  TranslationROffsetUnits=m  TranslationThetaOffset=0  TranslationThetaOffsetUnits=deg  TranslationZOffset=0  TranslationZOffsetUnits=m
  Transform Sensor : sm_lib/Frames and Transforms/Transform Sensor  MeasurementFrame=World  RotationSequence=XYX  SenseAngle=off  SenseAxis=off  SenseQ=off  SenseR=off  SenseRotationSequence=off  SenseOmegaX=off  SenseOmegaY=off  SenseOmegaZ=off  SenseOmega=off  SenseQDot=off  SenseRDot=off  SenseRotationSequenceDot=off  SenseAlphaX=off  SenseAlphaY=off  SenseAlphaZ=off  SenseAlpha=off  SenseQDDot=off  SenseRDDot=off  SenseX=on  SenseY=on  SenseZ=on  SenseXYZ=off  SenseRad=off  SenseAzim=off  SenseDist=off  SenseInc=off  SenseXDot=off  SenseYDot=off  SenseZDot=off  SenseXYZDot=off  SenseRadDot=off  SenseAzimDot=off  SenseDistDot=off  SenseIncDot=off  SenseXDDot=off  SenseYDDot=off  SenseZDDot=off  SenseXYZDDot=off  SenseRadDDot=off  SenseAzimDDot=off  SenseDistDDot=off  SenseIncDDot=off
  x : Constant  Value=129.3
  F : PMIOPort  Side=Left
  Wrld : PMIOPort  Port=2  Side=Right
  Out1 : Outport  VectorParamsAs1DForOutWhenUnconnected=off
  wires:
  Gain1/1 -> Terminator1/1  "y (mm)"
  PS-Simulink Converter2/1 -> Gain2/1
  x/1 -> Add/2
  Add/1 -> Scope/1, Out1/1, [Z], Terminator2/1  "z (mm)"
  PS-Simulink Converter1/1 -> Gain1/1
  Gain2/1 -> Add/1
  PS-Simulink Converter/1 -> Gain/1
  Gain/1 -> Terminator/1  "x (mm)"
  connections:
  Solid/RConn1 -- ReferenceFrame/RConn1 -- Transform Sensor/RConn1 -- Transform/LConn1
  Transform/RConn1 -- F/RConn1
  PS-Simulink Converter2/LConn1 -- Transform Sensor/RConn4
  Transform Sensor/RConn3 -- PS-Simulink Converter1/LConn1
  Transform Sensor/RConn2 -- PS-Simulink Converter/LConn1
  Wrld/RConn1 -- Transform Sensor/LConn1
